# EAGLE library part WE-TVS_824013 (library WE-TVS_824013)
TVS Diode Array WE-TVS, High Speed Series - Low capazity - No leakage current - Low clamping voltage - high ESD voltage protection -- 3.3 VDC Application
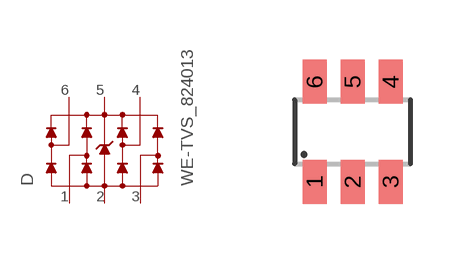
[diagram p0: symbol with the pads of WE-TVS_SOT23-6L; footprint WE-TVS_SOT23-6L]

Designator prefix D

## WE-TVS_824013 (MPN: 824013; OC_FARNELL: 1825869; OC_NEWARK: 79R6950; PACKAGE: SOT23-6L; SUPPLIER: Wuerth Elektronik)  [WE-TVS_SOT23-6L]
1  1  pas
2  GND  pwr
3  2  pas
4  3  pas
5  VDD  pwr
6  4  pas

## Footprint WE-TVS_SOT23-6L (pad centres in mm)
TVS Diode Array WE-TVS
smd 0.6 x 1.1: 1 -0.95,-1.25; 2 0,-1.25; 3 0.95,-1.25; 4 0.95,1.25; 5 0,1.25; 6 -0.95,1.25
